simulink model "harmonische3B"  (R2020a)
settings: Solver=ode45  StartTime=-8  StopTime=8  MaxStep=0.01  RelTol=1e-3  EnableMultiTasking=on

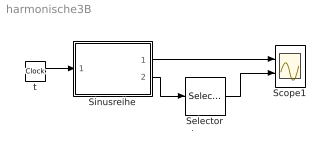
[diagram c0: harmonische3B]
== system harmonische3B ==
  note: .
  Scope1 : Scope  NumInputPorts=2
  Selector : Selector  IndexOptions=Index vector (dialog)  Indices=1:5  OutputSizes=1
  Sinusreihe : Subsystem  mask(Fouriersinus){Nh=1:50, bi=1./(1:50), A=2/pi}
      mask prompts: Nh "Nummern der Harmonischen"; bi "Koeffizienten der Harmonischen"; A "Skalierungsfaktor"
      mask help: Funktion, definiert als Fourierreihe mit Sinus Eingang: Argument Ausgang: Funktionswert und Vektor der Harmonischen
  t : Clock
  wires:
  Sinusreihe/1(y) -> Scope1/1
  t/1 -> Sinusreihe/1(t)
  Selector/1 -> Scope1/2
  Sinusreihe/2(harm) -> Selector/1

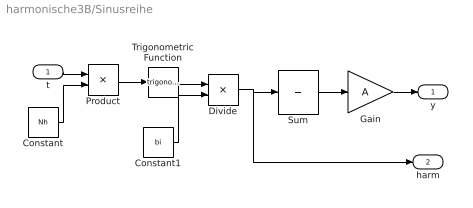
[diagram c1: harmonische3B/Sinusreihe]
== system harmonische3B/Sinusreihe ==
  t : Inport
  Constant : Constant  Value=Nh
  Constant1 : Constant  Value=bi
  Divide : Product
  Gain : Gain  Gain=A  SaturateOnIntegerOverflow=on
  Product : Product  RndMeth=Zero
  Sum : Sum  Inputs=+  SaturateOnIntegerOverflow=on
  Trigonometric Function : Trigonometry
  y : Outport
  harm : Outport  Port=2
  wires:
  Sum/1 -> Gain/1
  Divide/1 -> Sum/1, harm/1
  Constant/1 -> Product/2
  Product/1 -> Trigonometric Function/1
  Trigonometric Function/1 -> Divide/1
  t/1 -> Product/1
  Gain/1 -> y/1
  Constant1/1 -> Divide/2
